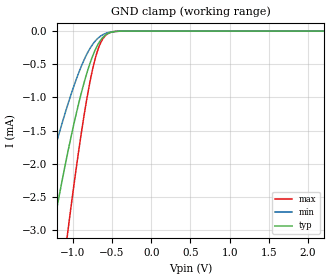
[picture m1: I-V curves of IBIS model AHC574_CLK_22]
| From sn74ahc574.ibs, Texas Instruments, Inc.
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[Model]   AHC574_CLK_22
Model_type  Input
Vinl = 0.5
Vinh = 1.5
| variable   typ   min   max
C_comp   0.87pF   0.75pF   1.03pF
[Temperature Range]   40   100   -40
| Ambient temperature   25   85   -40
[Voltage range]   2.2   2   2.4
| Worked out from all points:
|   GND clamp passes 1 mA (typ) near -0.91 V on its own axis
[GND Clamp]
| AHC574_CLK_22
|   Voltage   I(typ)   I(min)   I(max)
-2.2V     -10.52mA   -6.823mA   -15.45mA
-1.52V    -4.862mA   -3.106mA   -7.679mA
-1.49V    -4.639mA   -2.96mA    -7.353mA
-1.255V   -2.995mA   -1.878mA   -4.879mA
-1.065V   -1.826mA   -1.107mA   -3.025mA
-915mV    -1.038mA   -596.1uA   -1.716mA
-810mV    -588.3uA   -320.7uA   -941.5uA
-720mV    -296.9uA   -157.5uA   -437.3uA
-625mV    -105uA     -58.99uA   -130.7uA
-545mV    -32.01uA   -20.15uA   -32.37uA
-420mV    -3.333uA   -2.298uA   -2.129uA
2.2V      1.186nA    443.4pA    2.106nA
